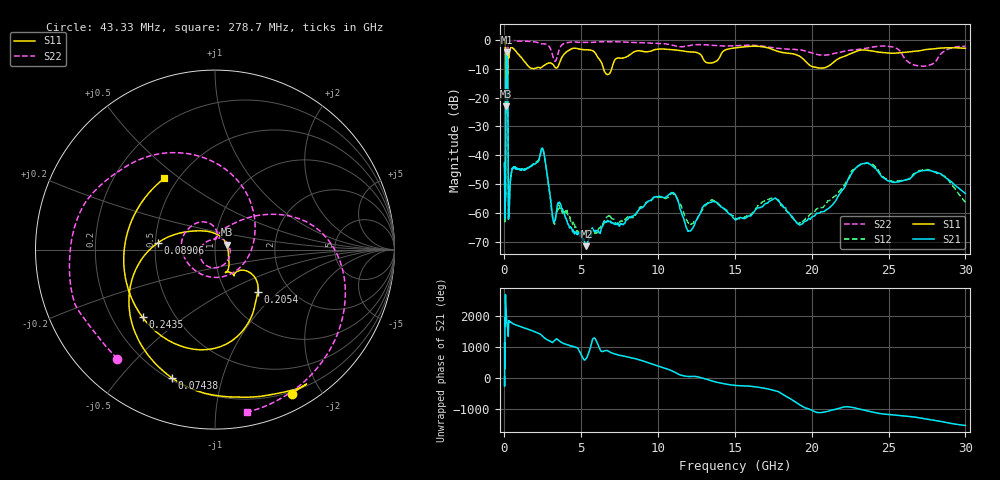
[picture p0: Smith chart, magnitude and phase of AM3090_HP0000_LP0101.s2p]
! Date/Time: Thu, Feb 28, 2019 1:53 PM
! Network Analyzer: Agilent Technologies E8364B Rev: A.07.50.67
! Sweep from 0.010 to 30.000 GHz, 1601 Points, Sweep Type: LOG
! Power Supply: 5.023 V, 0.002 A
# Hz S DB R 50
!freq MagS11 AngS11 MagS21 AngS21 MagS12 AngS12 MagS22 AngS22
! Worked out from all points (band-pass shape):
!   1601 points, 10 MHz to 30 GHz, reference 50 ohm
!   highest |S21| = -4.30 dB at 143.3 MHz (marker M1); lowest = -71.5 dB at 5.338 GHz (marker M2)
!   |S21| within 3 dB of the highest: 98.8 MHz to 201.1 MHz (102.3 MHz wide, 68.2 % of centre)
!   lowest |S11| = -23.0 dB at 97.46 MHz (marker M3), VSWR 1.15, Z = 56.9 + j3.13 ohm
!   |S11| at or under -10 dB: 89.16 MHz to 202.5 MHz (113.3 MHz wide, 77.7 % of centre); 6.455 GHz to 6.979 GHz (523.6 MHz wide, 7.8 % of centre)
!   |S22| runs from -25.2 to -0.1 dB; largest |S21 - S12| = 0.013
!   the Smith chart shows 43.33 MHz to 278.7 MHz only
!   S11 on the Smith chart (normalised r, x): 43.33 MHz: 0.18, -1.66; 74.38 MHz: 0.21, -0.70; 89.06 MHz: 0.51, +0.04; 205.4 MHz: 1.39, -0.75; 243.5 MHz: 0.33, -0.36; 278.7 MHz: 0.42, +0.44
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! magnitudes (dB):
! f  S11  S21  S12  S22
! 10 MHz  -0.3  -44.3  -44.0  -0.6
! 38.04 MHz  -0.5  -60.8  -60.9  -1.4
! 43.33 MHz  -0.8  -60.6  -60.2  -1.8
! 48.61 MHz  -0.9  -47.6  -49.9  -1.6
! 74.38 MHz  -2.5  -44.4  -46.0  -4.4
! 89.06 MHz  -9.9  -15.4  -15.4  -15.9
! 97.46 MHz  -23.0  -7.8  -7.8  -14.3
! 143.3 MHz  -15.3  -4.3  -4.3  -21.9
! 144.7 MHz  -15.2  -4.3  -4.3  -21.7
! 205.4 MHz  -9.5  -8.3  -8.2  -16.6
! 243.5 MHz  -5.2  -52.3  -51.6  -1.7
! 278.7 MHz  -6.2  -60.5  -61.7  -0.7
! 550.5 MHz  -2.9  -44.5  -44.4  -0.2
! 2.084 GHz  -9.7  -42.5  -42.2  -0.8
! 2.507 GHz  -9.1  -37.9  -38.1  -1.3
! 3.188 GHz  -8.6  -62.9  -63.1  -6.4
! 5.338 GHz  -3.4  -71.5  -66.2  -0.8
! 7.926 GHz  -5.9  -62.5  -61.8  -0.8
! 10.7 GHz  -3.3  -53.7  -54.4  -1.5
! 19.61 GHz  -7.5  -62.9  -61.9  -3.8
! 23.48 GHz  -3.5  -42.8  -42.8  -2.9
! 30 GHz  -2.9  -53.2  -56.4  -2.2
